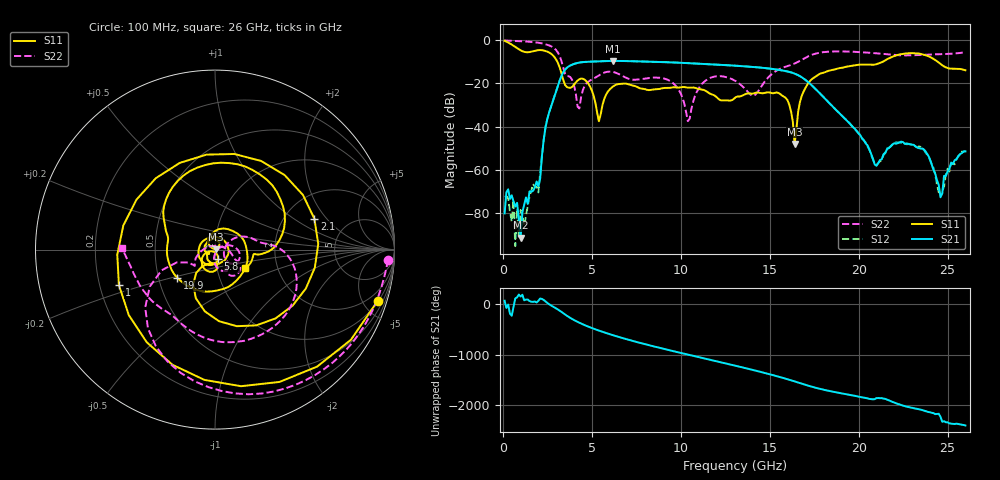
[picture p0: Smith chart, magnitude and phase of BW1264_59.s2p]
!Keysight Technologies,N5245B,MY57181159,A.13.60.06
!Date: Friday, December 18, 2020 23:55:09
!Correction: S11(Full 2 Port(1,2))
!S21(Full 2 Port(1,2))
!S12(Full 2 Port(1,2))
!S22(Full 2 Port(1,2))
!S2P File: Measurements: S11, S21, S12, S22:
# Hz S  dB  R 50
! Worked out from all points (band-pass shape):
!   260 points, 100 MHz to 26 GHz, reference 50 ohm
!   highest |S21| = -9.74 dB at 6.2 GHz (marker M1); lowest = -91.2 dB at 1 GHz (marker M2)
!   |S21| within 3 dB of the highest: 3.621 GHz to 14.4 GHz (10.78 GHz wide, 120 % of centre)
!   lowest |S11| = -48.1 dB at 16.4 GHz (marker M3), VSWR 1.01, Z = 50.3 + j0.215 ohm
!   |S11| at or under -10 dB: 3.053 GHz to 21.39 GHz (18.33 GHz wide, 150 % of centre); 24.42 GHz to end of sweep
!   |S22| runs from -37.5 to -0.3 dB; largest |S21 - S12| = 0.00066
!   S11 on the Smith chart (normalised r, x): 100 MHz: 1.07, -6.29; 1 GHz: 0.28, -0.17; 2.1 GHz: 2.90, +1.51; 5.8 GHz: 1.03, -0.11; 19.9 GHz: 0.63, -0.21; 26 GHz: 1.37, -0.30
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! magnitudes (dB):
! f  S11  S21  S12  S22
! 100 MHz  -0.4  -80.1  -72.5  -0.3
! 1 GHz  -4.9  -91.2  -78.5  -0.6
! 2.1 GHz  -4.7  -63.9  -61.4  -1.5
! 2.4 GHz  -5.2  -40.3  -40.2  -2.1
! 3.2 GHz  -12.8  -18.7  -18.7  -7.6
! 4.2 GHz  -18.8  -10.7  -10.7  -30.8
! 4.5 GHz  -18.0  -10.3  -10.3  -23.1
! 5.4 GHz  -37.6  -9.9  -9.9  -16.4
! 5.8 GHz  -25.3  -9.8  -9.8  -14.9
! 6.2 GHz  -21.5  -9.7  -9.7  -14.8
! 8.8 GHz  -22.7  -10.2  -10.2  -17.5
! 10.4 GHz  -22.1  -10.8  -10.7  -37.5
! 11.4 GHz  -23.6  -11.2  -11.2  -18.8
! 13.1 GHz  -26.4  -12.0  -12.0  -19.1
! 15.9 GHz  -26.8  -14.4  -14.4  -12.4
! 16.4 GHz  -48.1  -15.6  -15.6  -10.9
! 17.4 GHz  -18.0  -21.3  -21.3  -6.8
! 19.9 GHz  -11.6  -42.2  -42.1  -5.6
! 21.7 GHz  -8.6  -49.9  -49.8  -6.8
! 23.7 GHz  -7.0  -50.8  -51.2  -6.9
! 24.6 GHz  -11.1  -72.6  -70.4  -6.6
! 26 GHz  -14.1  -51.5  -51.3  -5.7
